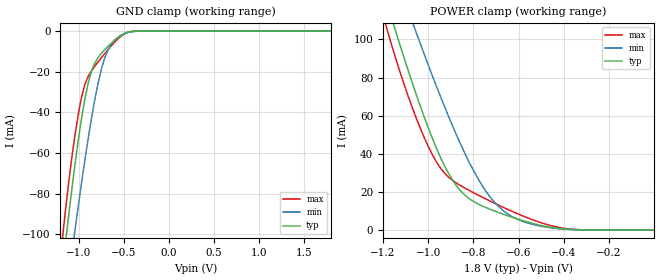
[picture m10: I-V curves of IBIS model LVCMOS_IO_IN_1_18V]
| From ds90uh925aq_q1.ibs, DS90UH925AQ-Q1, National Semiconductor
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[Model] LVCMOS_IO_IN_1_18V
Model_type Input
Vinh = 0.0V
Vinl = 0.0V
C_comp   3.52pF   2.88pF   4.05pF
[Voltage Range]   1.8V   1.62V   1.98V
[Temperature Range]   25.0   130.0   -40.0
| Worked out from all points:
|   GND clamp passes 1 mA (typ) near -0.48 V on its own axis
|   POWER clamp passes 1 mA (typ) near -0.44 V on its own axis
[GND Clamp]
-1.8V     -382.9mA   -371.7mA   -403.9mA
-1.184V   -120.1mA   -147.5mA   -104.8mA
-1.147V   -105.2mA   -134.4mA   -89.12mA
-1.114V   -92.76mA   -123.2mA   -76.53mA
-1.039V   -65.46mA   -97.83mA   -51.04mA
-968.4mV  -43.41mA   -75.34mA   -32.92mA
-892.8mV  -25.56mA   -52.82mA   -22.28mA
-822.6mV  -16.01mA   -34.38mA   -17.48mA
-747mV    -10.95mA   -18.74mA   -13.14mA
-639mV    -6.024mA   -6.586mA   -7.366mA
-531mV    -2.173mA   -2.121mA   -2.558mA
1.796V    905.6pA    0A         -53.48pA
[POWER Clamp]
-1.8V     378.8mA    370.5mA    398.3mA
-1.179V   117.8mA    145.8mA    104mA
-1.141V   103.3mA    133mA      89.12mA
-1.055V   71.83mA    104.3mA    59.38mA
-963mV    42.81mA    75.32mA    35.62mA
-925.2mV  33.13mA    64.06mA    29.51mA
-871.2mV  22.64mA    48.92mA    24.34mA
-763.2mV  12.73mA    23.71mA    17.38mA
-671.4mV  8.429mA    10.49mA    12.09mA
-563.4mV  4.296mA    3.787mA    6.539mA
-401.4mV  516.5uA    499.6uA    897.2uA
-1.8mV    1.16nA     23.5nA     127.3pA
